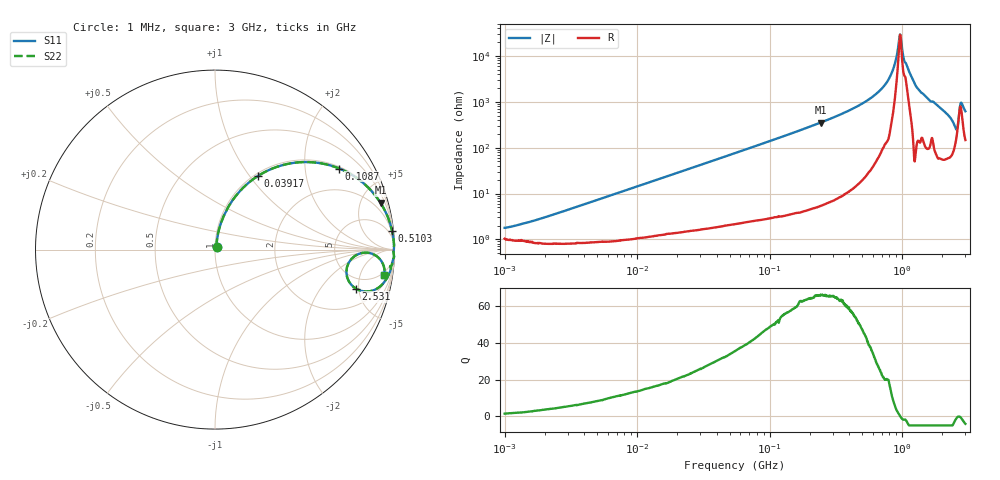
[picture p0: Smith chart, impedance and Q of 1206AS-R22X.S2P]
!s-Parameter Generated by FASTRON Sdn. Bhd.
!FASTRON P/N : 1206AS-R22X
!Keysight Technologies: E4991B_MY54100416_A.01.15
!Date created: Thu Nov 16 10:07:09 2023
!Version  : Rev00 Thu Nov 16 10:07:09 2023
!Data & Calibration Information:
!Freq	S11	S21	S12	S22
!PortZ  Port1:50+j0  Port2:50+j0
!When reading reference impedance value at option line is always used.
! Remarks : This data is being provided solely for informational purposes.
# Hz S dB R 50
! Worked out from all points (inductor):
!   1601 points, 1 MHz to 3 GHz, reference 50 ohm
!   read as one part in series: L = 230 nH near 1.717 MHz
!   highest Q = 65.9 at 242.1 MHz (marker M1), where L = 232 nH
!   self-resonance near 963.4 MHz
!   S11 on the Smith chart (normalised r, x): 1 MHz: 1.02, +0.03; 39.17 MHz: 1.04, +1.09; 108.7 MHz: 1.06, +3.03; 510.3 MHz: 1, +19; 2.531 GHz: 3.59, -4.68; 3 GHz: 4, -12
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1000000  -35.08 53.8  -0.09 -0.8  -0.09 -0.8  -35.08 53.8
3804036  -25.20 78.3  -0.08 -3.1  -0.08 -3.1  -25.20 78.3
1.447069e7  -14.05 75.2  -0.28 -11.4  -0.28 -11.4  -14.05 75.2
3.917023e7  -6.51 59.9  -1.25 -28.2  -1.25 -28.2  -6.51 59.9
5.477226e7  -4.47 51.7  -2.10 -36.7  -2.10 -36.7  -4.47 51.7
1.087149e8  -1.65 33.1  -5.25 -55.7  -5.25 -55.7  -1.65 33.1
2.083556e8  -0.50 18.4  -10.00 -70.7  -10.00 -70.7  -0.50 18.4
2.421036e8  -0.37 15.8  -11.31 -73.4  -11.31 -73.4  -0.37 15.8
5.102796e8  -0.07 6.0  -19.63 -82.8  -19.63 -82.8  -0.07 6.0
6.685918e8  -0.03 3.4  -24.63 -84.5  -24.63 -84.5  -0.03 3.4
7.925923e8  -0.02 1.8  -30.00 -85.2  -30.00 -85.2  -0.02 1.8
8.629671e8  -0.02 1.0  -34.96 -81.5  -34.96 -81.5  -0.02 1.0
9.395906e8  -0.03 0.3  -45.23 -54.2  -45.23 -54.2  -0.03 0.3
9.682285e8  -0.03 -0.0  -49.32 4.7  -49.32 4.7  -0.03 -0.0
1.059487e9  -0.06 -0.7  -37.15 61.4  -37.15 61.4  -0.06 -0.7
1.294266e9  -0.04 -2.8  -26.23 83.7  -26.23 83.7  -0.04 -2.8
2.177892e9  -0.30 -10.1  -15.04 73.8  -15.04 73.8  -0.30 -10.1
2.530652e9  -1.77 -15.5  -10.30 45.6  -10.30 45.6  -1.77 -15.5
2.594767e9  -2.58 -9.7  -10.58 25.0  -10.58 25.0  -2.58 -9.7
2.673854e9  -1.70 -1.3  -14.96 5.8  -14.96 5.8  -1.70 -1.3
2.783064e9  -0.67 -3.7  -20.30 37.8  -20.30 37.8  -0.67 -3.7
3e9  -0.42 -8.5  -16.33 67.9  -16.33 67.9  -0.42 -8.5
